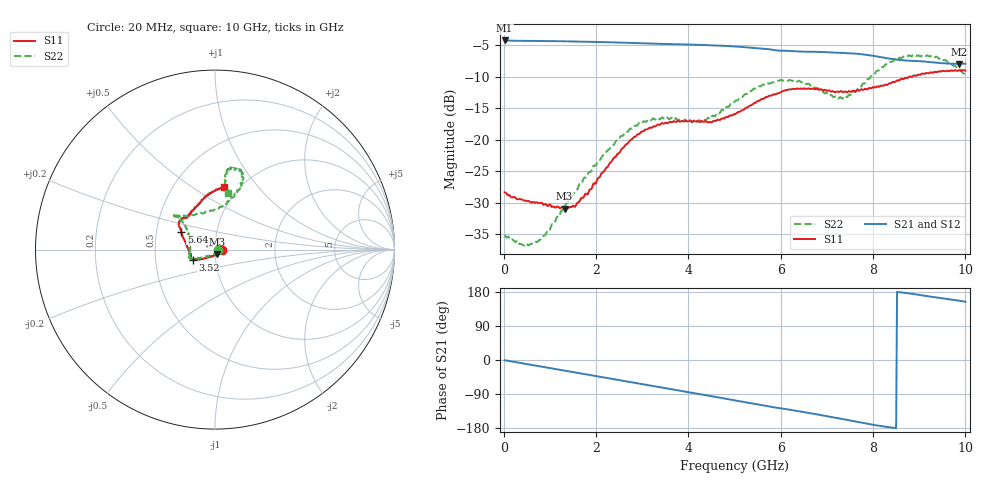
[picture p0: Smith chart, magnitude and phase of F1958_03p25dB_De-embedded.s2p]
! Integrated Device Technology
! Corporate Headquarters
! 6024 Silver Creek Valley Road
! San Jose, CA 95138  USA
! Phone:  1-408-284-8200
! Toll Free:  1-800-223-1366
! Webpage:  http://www.idt.com/
! Timing and RF Division
! 515 Groton Road, Suite 102
! Westford, MA 01886-6024
! Device:  F1958
! Description: 7-bit 0.25 dB Digital Step Attenuator
! Frequency:  0.001 -  6.000 GHz
! Package:  4x4 mm Thin QFN Plastic Package: 24 pin
! Ports:  2 RF, 12 DC
!  Pin  1  = D0
!  Pin  2  = VDD
!  Pin  3  = VMODE
!  Pin  4  = GND
!  Pin  5  = RF1  =  Port 1
!  Pin  6  = GND
!  Pin  7  = GND
!  Pin  8  = GND
!  Pin  9  = GND
!  Pin 10  = GND
!  Pin 11  = GND
!  Pin 12  = GND
!  Pin 13  = GND
!  Pin 14  = RF2  =  Port 2
!  Pin 15  = GND
!  Pin 16  = LE
!  Pin 17  = CLK
!  Pin 18  = DATA
!  Pin 19  = D6
!  Pin 20  = D5
!  Pin 21  = D4
!  Pin 22  = D3
!  Pin 23  = D2
!  Pin 24  = D1
! State:  13
! Atten State:  3.25 dB
! Voltage:  +3.30 Volts
! Current:  0.258 mA
! Data:  The device was measured on a F1958 evaluation board which has
!  individual transmission lines to the RF pins.  Data was collected
!  using a calibrated network analyzer.  The evaluation board was
!  de-embedded using Automatic Fixture Removal (AFR).
!  The reference plane is the edge of the package pin.
! Misc:
!  Action Tracker AT0419
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# GHz S dB R 50
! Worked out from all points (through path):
!   500 points, 20 MHz to 10 GHz, reference 50 ohm
!   highest |S21| = -4.26 dB at 20 MHz (marker M1); lowest = -8.0 dB at 9.86 GHz (marker M2)
!   group delay of S21, straight-line fit = 58.2 ps
!   lowest |S11| = -30.9 dB at 1.32 GHz (marker M3), VSWR 1.06, Z = 51.1 - j2.66 ohm
!   |S11| at or under -10 dB: start of sweep to 8.786 GHz; 8.810371 GHz to 8.847795 GHz (37.42 MHz wide, 0.424 % of centre)
!   |S22| runs from -36.9 to -6.6 dB; largest |S21 - S12| = 0.0015
!   S11 on the Smith chart (normalised r, x): 20 MHz: 1.08, -0.00; 3.52 GHz: 0.77, -0.09; 5.64 GHz: 0.67, +0.14; 10 GHz: 0.86, +0.69
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0.02  -28.35 -3.2  -4.26 -0.6  -4.26 -0.5  -35.10 -6.9
0.44  -29.63 -11.6  -4.33 -9.5  -4.33 -9.4  -36.81 -33.0
0.7  -29.93 -21.6  -4.34 -14.9  -4.34 -14.9  -36.18 -54.3
0.96  -30.51 -35.5  -4.36 -20.4  -4.36 -20.4  -34.29 -80.0
1.32  -30.92 -66.4  -4.40 -28.1  -4.40 -28.1  -30.67 -113.8
1.52  -30.54 -83.6  -4.43 -32.3  -4.42 -32.3  -28.49 -125.4
1.7  -29.19 -98.2  -4.45 -36.1  -4.45 -36.0  -26.75 -133.5
2.58  -21.32 -142.0  -4.61 -54.8  -4.60 -54.8  -19.37 -152.5
2.94  -19.06 -150.0  -4.69 -62.4  -4.68 -62.5  -17.35 -156.2
3.36  -17.61 -154.7  -4.79 -71.3  -4.80 -71.4  -16.66 -160.4
3.52  -17.30 -156.0  -4.82 -74.7  -4.82 -74.8  -16.49 -164.6
4.32  -17.16 -166.7  -4.98 -91.7  -4.99 -91.7  -16.76 167.8
5.02  -15.91 170.8  -5.22 -106.8  -5.23 -106.8  -13.81 143.1
5.64  -13.44 152.0  -5.56 -120.2  -5.58 -120.2  -11.28 139.1
6.18  -12.02 143.7  -5.92 -130.9  -5.94 -130.8  -10.56 139.9
6.68  -11.90 137.2  -6.06 -141.1  -6.08 -141.0  -11.45 135.0
7.38  -12.35 128.6  -6.25 -156.7  -6.25 -156.6  -13.13 96.8
8.34  -11.10 106.7  -7.12 -177.4  -7.13 -177.5  -7.93 67.7
8.76  -10.15 95.7  -7.47 175.9  -7.47 176.0  -6.67 71.1
9.24  -9.33 86.0  -7.70 167.2  -7.70 167.2  -6.79 78.7
9.86  -9.00 81.2  -7.97 156.6  -8.00 156.6  -8.83 79.8
10  -9.04 81.4  -7.94 153.5  -7.97 153.7  -9.76 77.2
